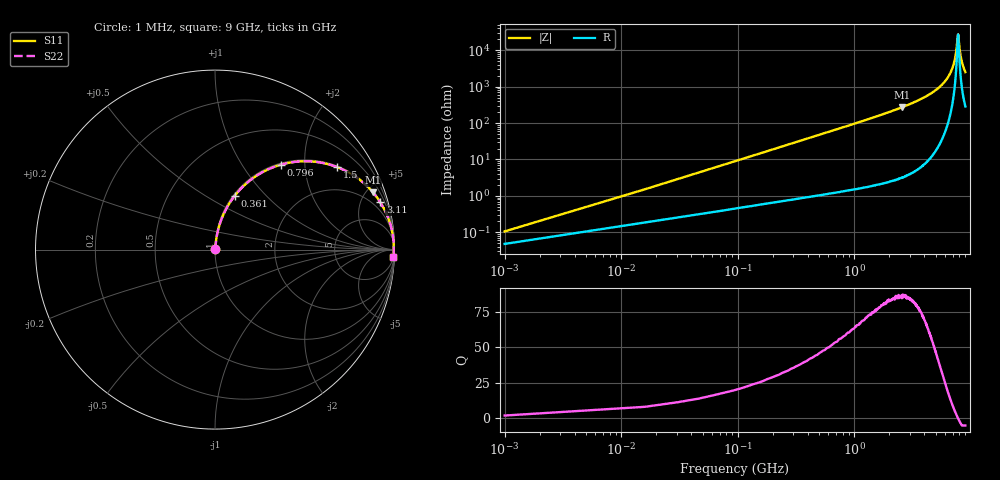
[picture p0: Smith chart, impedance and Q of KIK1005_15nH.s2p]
!version-3
!date-01.2023
!Series
# MHz S RI R 50
!Freq ReS11 ImS11 ReS21 ImS21 ReS12 ImS12 ReS22 ImS22
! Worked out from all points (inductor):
!   601 points, 1 MHz to 9 GHz, reference 50 ohm
!   read as one part in series: L = 15 nH near 46 MHz
!   highest Q = 86 at 2.58 GHz (marker M1), where L = 16.9 nH
!   self-resonance near 7.79 GHz
!   S11 on the Smith chart (normalised r, x): 1 MHz: 1.00, +0.00; 361 MHz: 1.02, +0.68; 796 MHz: 1.03, +1.52; 1.5 GHz: 1.04, +2.94; 3.11 GHz: 1.08, +6.96; 9 GHz: 7, -50
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1  0.00046 0.000942  0.9995 -0.000942  0.9995 -0.000942  0.00046 0.000942
61  0.00683 0.0569  0.9932 -0.0569  0.9932 -0.0569  0.00683 0.0569
91  0.0116 0.0844  0.9884 -0.0844  0.9884 -0.0844  0.0116 0.0844
196  0.0388 0.1765  0.9612 -0.1765  0.9612 -0.1765  0.0388 0.1765
361  0.1103 0.3007  0.8897 -0.3007  0.8897 -0.3007  0.1103 0.3007
796  0.3673 0.4734  0.6327 -0.4734  0.6327 -0.4734  0.3673 0.4734
1500  0.6812 0.4594  0.3188 -0.4594  0.3188 -0.4594  0.6812 0.4594
1520  0.6858 0.4577  0.3142 -0.4577  0.3142 -0.4577  0.6858 0.4577
2580  0.8791 0.3203  0.1209 -0.3203  0.1209 -0.3203  0.8791 0.3203
3020  0.9152 0.2727  0.0848 -0.2727  0.0848 -0.2727  0.9152 0.2727
3110  0.9211 0.2636  0.0789 -0.2636  0.0789 -0.2636  0.9211 0.2636
4520  0.9738 0.1514  0.0262 -0.1514  0.0262 -0.1514  0.9738 0.1514
6020  0.9922 0.0703  0.00783 -0.0703  0.00783 -0.0703  0.9922 0.0703
6980  0.9959 0.0298  0.00412 -0.0298  0.00412 -0.0298  0.9959 0.0298
7280  0.9963 0.0184  0.00372 -0.0184  0.00372 -0.0184  0.9963 0.0184
7520  0.9964 0.00958  0.00361 -0.00958  0.00361 -0.00958  0.9964 0.00958
7740  0.9964 0.0016  0.00365 -0.0016  0.00365 -0.0016  0.9964 0.0016
7800  0.9963 -0.000486  0.00368 0.000486  0.00368 0.000486  0.9963 -0.000486
8040  0.9961 -0.00868  0.00391 0.00868  0.00391 0.00868  0.9961 -0.00868
8250  0.9958 -0.0156  0.00421 0.0156  0.00421 0.0156  0.9958 -0.0156
8580  0.9951 -0.0262  0.00489 0.0262  0.00489 0.0262  0.9951 -0.0262
9000  0.994 -0.0391  0.00605 0.0391  0.00605 0.0391  0.994 -0.0391
